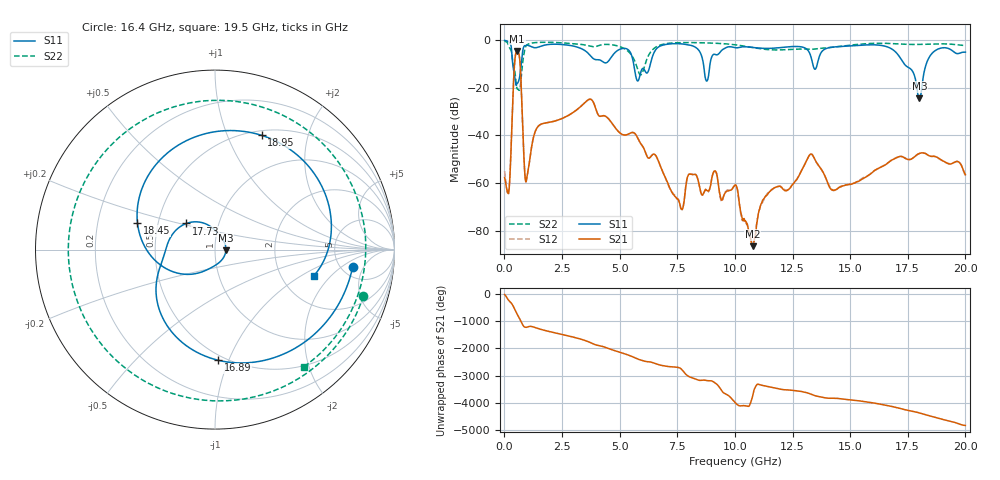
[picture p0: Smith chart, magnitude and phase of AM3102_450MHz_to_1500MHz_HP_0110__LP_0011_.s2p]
!Agilent Technologies,E8364B,MY43040894,A.07.50.67
!Agilent E8364B: A.07.50.67
!Date: Thursday, January 11, 2018 05:46:20
!Correction: S11(Full 2 Port(1,2))
!S21(Full 2 Port(1,2))
!S12(Full 2 Port(1,2))
!S22(Full 2 Port(1,2))
!S2P File: Measurements: S11, S21, S12, S22:
# Hz S  dB  R 50
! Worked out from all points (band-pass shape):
!   1601 points, 10 MHz to 20 GHz, reference 50 ohm
!   highest |S21| = -4.54 dB at 547.2 MHz (marker M1); lowest = -86.5 dB at 10.78 GHz (marker M2)
!   |S21| within 3 dB of the highest: 463.3 MHz to 660.8 MHz (197.5 MHz wide, 35.1 % of centre)
!   lowest |S11| = -24.3 dB at 18 GHz (marker M3), VSWR 1.13, Z = 56.5 - j0.321 ohm
!   |S11| at or under -10 dB: 363.2 MHz to 731.6 MHz (368.4 MHz wide, 67.3 % of centre); 5.61 GHz to 6.332 GHz (722.5 MHz wide, 12.1 % of centre); 17.35 GHz to 18.3 GHz (949.1 MHz wide, 5.32 % of centre)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
!   |S22| runs from -21.0 to -0.4 dB; largest |S21 - S12| = 0.0012
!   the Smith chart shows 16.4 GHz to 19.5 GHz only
!   S11 on the Smith chart (normalised r, x): 16.4 GHz: 6.29, -3.06; 16.89 GHz: 0.46, -0.92; 17.73 GHz: 0.70, +0.21; 18.45 GHz: 0.38, +0.14; 18.95 GHz: 0.55, +1.34; 19.5 GHz: 3.04, -1.31
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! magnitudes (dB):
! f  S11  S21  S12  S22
! 10 MHz  -0.1  -57.7  -55.0  -0.4
! 197.4 MHz  -0.7  -63.1  -63.0  -2.5
! 547.2 MHz  -18.1  -4.5  -4.5  -20.3
! 959.5 MHz  -2.0  -58.6  -58.7  -2.2
! 1.459 GHz  -2.9  -36.2  -36.2  -0.9
! 3.346 GHz  -3.5  -27.5  -27.5  -1.7
! 6.682 GHz  -2.8  -50.7  -50.8  -2.3
! 7.681 GHz  -1.5  -71.1  -71.0  -1.0
! 8.781 GHz  -17.1  -63.1  -63.6  -1.1
! 10.01 GHz  -3.1  -60.9  -61.1  -1.9
! 10.78 GHz  -3.0  -86.5  -84.9  -3.0
! 13.34 GHz  -8.4  -47.9  -47.9  -3.8
! 14.28 GHz  -2.8  -63.1  -63.2  -2.9
! 16.4 GHz  -2.2  -53.0  -53.0  -1.2
! 16.68 GHz  -3.0  -51.2  -51.2  -1.3
! 16.89 GHz  -4.2  -49.9  -49.8  -1.4
! 17.73 GHz  -13.3  -49.5  -49.5  -1.7
! 18 GHz  -24.3  -47.6  -47.5  -1.7
! 18.45 GHz  -6.8  -48.7  -48.7  -1.6
! 18.95 GHz  -3.3  -50.3  -50.4  -1.5
! 19.5 GHz  -4.9  -51.4  -51.5  -1.7
! 20 GHz  -5.0  -56.5  -57.0  -2.2
